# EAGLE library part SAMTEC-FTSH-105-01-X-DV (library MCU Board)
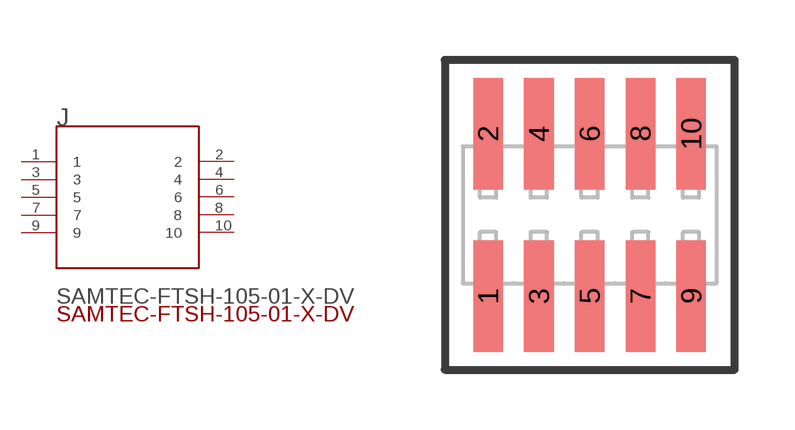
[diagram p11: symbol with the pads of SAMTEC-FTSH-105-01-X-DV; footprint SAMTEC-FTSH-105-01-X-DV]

Designator prefix J

## SAMTEC-FTSH-105-01-X-DVJ  [SAMTEC-FTSH-105-01-X-DV]
1  1  pas
2  2  pas
3  3  pas
4  4  pas
5  5  pas
6  6  pas
7  7  pas
8  8  pas
9  9  pas
10  10  pas

## Footprint SAMTEC-FTSH-105-01-X-DV (pad centres in mm)
translated Allegro footprint
smd 0.74 x 2.79: 1 -2.54,-2.032; 2 -2.54,2.032; 3 -1.27,-2.032; 4 -1.27,2.032; 5 0,-2.032; 6 0,2.032; 7 1.27,-2.032; 8 1.27,2.032; 9 2.54,-2.032; 10 2.54,2.032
